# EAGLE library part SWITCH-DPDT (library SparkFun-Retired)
DPDT Version of the COM-00597
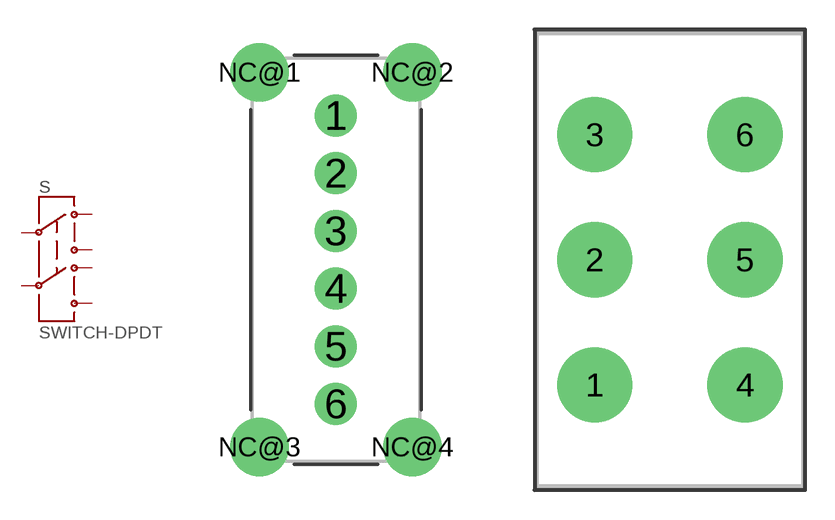
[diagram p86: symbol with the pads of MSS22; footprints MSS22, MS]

Designator prefix S

## SWITCH-DPDTPTH (PROD_ID: SWCH-09244)  [MSS22]
1  1
2  2
3  3
4  4
5  5
6  6

## SWITCH-DPDTPTH1 (SF_SKU: COM-11139)  [MS]
Pads as for MSS22

## SWITCH-DPDTES  [ES]
Pads as for MSS22

## SWITCH-DPDTOS  [OS]
Pads as for MSS22

## SWITCH-DPDTEG2211  [EG2211]
P1  2
P1-TA  1
P1-TB  3
P2  5
P2-TA  4
P2-TB  6

## SWITCH-DPDTSTOMP-PTH (PROD_ID: SWCH-12340; SF_SKU: COM-11151)  [STOMP-SWITCH-DPDT]
P$1  1
P$2  2
P$3  3
P$4  4
P$5  5
P$6  6

## Footprint MSS22 (pad centres in mm)
MSS22 DPDT Switch
drill 0.95: 1 2.65,11.5; 2 2.65,9.5; 3 2.65,7.5; 4 2.65,5.5; 5 2.65,3.5; 6 2.65,1.5
drill 1.35: NC@1 0,13; NC@2 5.3,13; NC@3 0,0; NC@4 5.3,0

## Footprint MS (pad centres in mm)
Series S Slide Switch
drill 2.8 pad 3.302: 1 -3.81,-6.35; 2 -3.81,0; 3 -3.81,6.35; 4 3.81,-6.35; 5 3.81,0; 6 3.81,6.35

## Footprint ES (pad centres in mm)
Right Angle Slide Switch. Works with part#ES21MABE
drill 0.864 pad 1.27: 1 2.54,2.54; 2 0,2.54; 3 -2.54,2.54; 4 2.54,0; 5 0,0; 6 -2.54,0
drill 0.9 pad 1.676: NC@1 -2.54,7.62; NC@2 2.54,7.62

## Footprint OS (pad centres in mm)
drill 0.787 pad 1.27: 1 -2.007,1.245; 2 0,1.245; 3 2.007,1.245; 4 -2.007,-1.245; 5 0,-1.245; 6 2.007,-1.245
